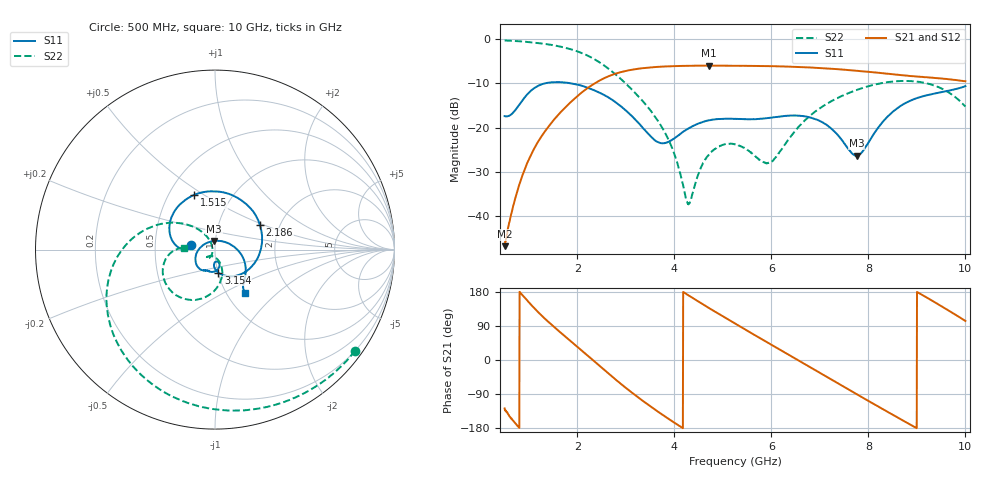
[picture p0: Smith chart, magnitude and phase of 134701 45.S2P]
!  2-Port S-parameters saved by WinCal
! VAR MeasName=S-Parameters (CALIBRATED_DATA) read from VNA (N5242A)
! VAR MeasDate=2013-7-3 16:38:13
! VAR NAME=134701 45
! VAR FILENAME=134701 45.S2P
! VAR DATE=2013-7-3 16:38:13
! VAR PHYS_PORTS=1,2
# Hz S MA R 50
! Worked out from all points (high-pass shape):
!   1601 points, 500 MHz to 10 GHz, reference 50 ohm
!   highest |S21| = -6.00 dB at 4.716 GHz (marker M1); lowest = -46.7 dB at 500 MHz (marker M2)
!   |S21| within 3 dB of the highest: 2.523 GHz to 9.593 GHz (7.07 GHz wide, 117 % of centre)
!   lowest |S11| = -26.3 dB at 7.756 GHz (marker M3), VSWR 1.10, Z = 49.2 + j4.73 ohm
!   |S11| at or under -10 dB: start of sweep to 1.335 GHz; 1.859 GHz to end of sweep
!   |S22| runs from -37.3 to -0.3 dB; largest |S21 - S12| = 0.0029
!   S11 on the Smith chart (normalised r, x): 500 MHz: 0.76, +0.04; 1.515 GHz: 0.67, +0.46; 2.186 GHz: 1.58, +0.47; 3.154 GHz: 1.00, -0.26; 10 GHz: 1.22, -0.64
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5e8  0.1349 170.2  0.004605 -127.7  0.004687 -129.0  0.9628 -35.9
7.196875e8  0.1575 179.7  0.01596 -166.4  0.01609 -166.7  0.9494 -51.4
9.334375e8  0.2262 172.3  0.036 162.0  0.03596 161.8  0.9308 -66.6
1.206562e9  0.2994 145.3  0.07176 124.5  0.07167 124.3  0.8981 -85.8
1.515312e9  0.3264 110.5  0.1225 87.9  0.1221 87.8  0.848 -107.8
2.085312e9  0.2974 41.6  0.2477 25.7  0.2472 25.6  0.6964 -149.1
2.18625e9  0.2852 28.5  0.2731 14.6  0.2724 14.6  0.6591 -156.6
2.643438e9  0.2187 -29.8  0.3802 -35.9  0.3802 -35.8  0.4613 172.0
3.154062e9  0.13 -81.6  0.4531 -89.0  0.4531 -89.0  0.2588 144.8
3.670625e9  0.06852 -88.0  0.4857 -137.1  0.4852 -137.1  0.1173 125.7
3.973438e9  0.07407 -74.4  0.494 -163.2  0.4938 -163.2  0.05498 120.1
4.282188e9  0.0973 -75.7  0.4984 171.3  0.4986 171.4  0.01391 178.8
4.715625e9  0.1211 -89.7  0.501 137.0  0.5009 137.0  0.0499 -122.5
5.25e9  0.1256 -105.3  0.4991 96.2  0.4993 96.1  0.06493 -134.7
5.956562e9  0.129 -115.5  0.4942 43.4  0.4939 43.4  0.04038 -102.2
6.395938e9  0.1368 -126.9  0.487 10.7  0.4874 10.6  0.07904 -69.3
6.835312e9  0.1283 -146.8  0.4763 -22.0  0.4764 -22.0  0.1421 -73.4
7.31625e9  0.08867 177.3  0.4588 -57.7  0.4581 -57.8  0.2099 -86.5
7.755625e9  0.04827 96.7  0.4378 -90.1  0.4374 -90.2  0.2657 -100.4
8.420625e9  0.1375 -5.9  0.4048 -138.6  0.4032 -138.6  0.3271 -124.7
9.16875e9  0.2292 -43.5  0.3703 167.4  0.3706 167.5  0.3198 -155.5
1e10  0.2939 -55.3  0.3338 103.0  0.3344 103.3  0.1727 176.8
